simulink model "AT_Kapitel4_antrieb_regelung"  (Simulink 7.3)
settings: Solver=ode15s  StartTime=0.0  StopTime=60  RelTol=1e-3
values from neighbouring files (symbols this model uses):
  c_T = .2e-1    (= 0.02)    [set_data.m]
  d_T = 0    [set_data.m]
  k_A = .9    (= 0.9)    [set_data.m]
  L_A = 3/200    (= 0.015)    [set_data.m]
  R_A = 20    [set_data.m]
  theta_G = .3500000000e-2    (= 0.0035)    [set_data.m]
  theta_L = .6300000000e-2    (= 0.0063)    [set_data.m]
  u_ZW = 200    [set_data.m]
libraries: cstblocks x2, simulink x1

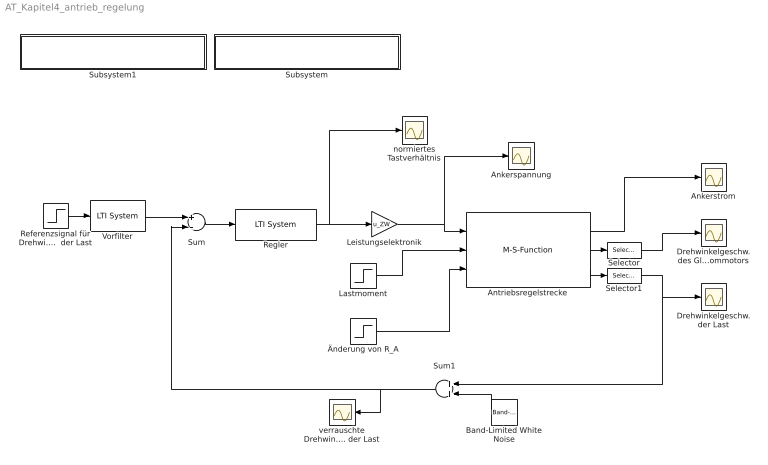
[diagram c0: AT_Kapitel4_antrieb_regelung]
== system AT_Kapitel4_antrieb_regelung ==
  Ankerspannung : Scope
  Ankerstrom : Scope
  Antriebsregelstrecke : M-S-Function  FunctionName=Antrieb_S_m  Parameters=RAp,LAp,kAp,thetaGp,thetaLp,cTp,dTp  mask{RAp=R_A, LAp=L_A, kAp=k_A, thetaGp=theta_G, thetaLp=theta_L, cTp=c_T, dTp=d_T}
      mask prompts: RAp "Ankerwiderstand"; LAp "Ankerinduktivität"; kAp "Ankerkreiskonstante"; thetaGp "Trägheitsmoment GSM"; thetaLp "Trägheitsmoment Last"; cTp "Federsteifigkeit"; dTp "Dämpfungskonstante"
  Band-Limited White Noise : simulink/Sources/Band-Limited White Noise  SystemSampleTime=-1  Cov=[0.2]  Ts=0.05  seed=[23341]
  Drehwinkelgeschw. der Last : Scope
  Drehwinkelgeschw. des Gleichstrommotors : Scope
  Lastmoment : Step  Time=20  SampleTime=0
  Leistungselektronik : Gain  Gain=u_ZW  ParameterDataType=sfix(16)  ParameterScaling=2^0  OutDataType=sfix(16)  OutScaling=2^0
  Referenzsignal für Drehwinkelgeschw.  der Last : Step  Time=10  Before=100  After=-100  SampleTime=0
  Regler : cstblocks/LTI System  SystemSampleTime=-1  sys=R  IC=[]
  Selector : Selector  InputPortWidth=2  IndexOptions=Index vector (dialog)  Indices=[2]  OutputSizes=1
  Selector1 : Selector  InputPortWidth=2  IndexOptions=Index vector (dialog)  Indices=[2]  OutputSizes=1
  Subsystem : Subsystem  Description=test
  Subsystem1 : Subsystem  Description=test
  Sum : Sum  Inputs=+-  OutDataType=sfix(16)  OutScaling=2^0
  Sum1 : Sum  OutDataType=sfix(16)  OutScaling=2^0
  Vorfilter : cstblocks/LTI System  SystemSampleTime=-1  sys=F  IC=[]
  normiertes Tastverhältnis : Scope
  verrauschte Drehwinkelgeschw. der Last : Scope
  Änderung von R_A : Step  Time=40  Before=1  After=1.4  SampleTime=0
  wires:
  Regler/1 -> normiertes Tastverhältnis/1, Leistungselektronik/1
  Sum/1 -> Regler/1
  Referenzsignal für Drehwinkelgeschw.  der Last/1 -> Vorfilter/1
  Vorfilter/1 -> Sum/1
  Sum1/1 -> Sum/2, verrauschte Drehwinkelgeschw. der Last/1
  Leistungselektronik/1 -> Antriebsregelstrecke/1, Ankerspannung/1
  Lastmoment/1 -> Antriebsregelstrecke/2
  Änderung von R_A/1 -> Antriebsregelstrecke/3
  Antriebsregelstrecke/1 -> Ankerstrom/1
  Antriebsregelstrecke/2 -> Selector/1
  Selector/1 -> Drehwinkelgeschw. des Gleichstrommotors/1
  Antriebsregelstrecke/3 -> Selector1/1
  Selector1/1 -> Drehwinkelgeschw. der Last/1, Sum1/1
  Band-Limited White Noise/1 -> Sum1/2

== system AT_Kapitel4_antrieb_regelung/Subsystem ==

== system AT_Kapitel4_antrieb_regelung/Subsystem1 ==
